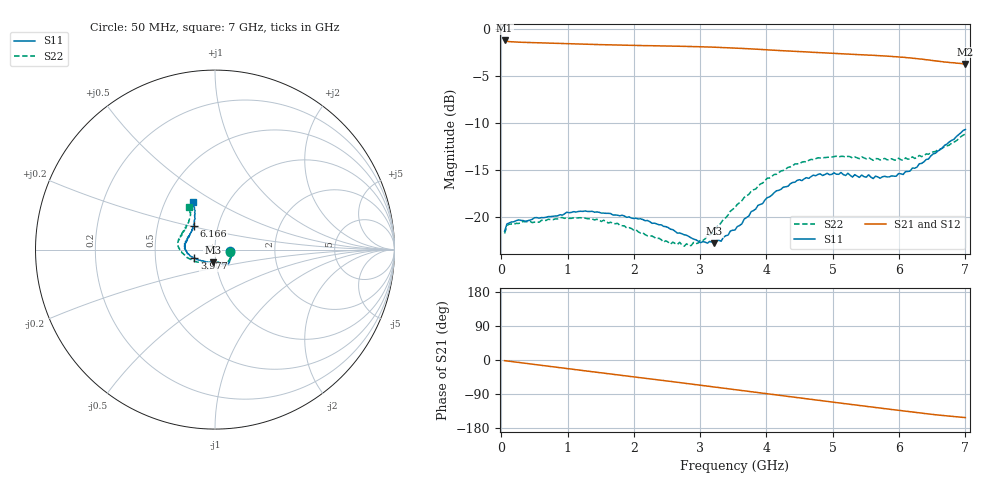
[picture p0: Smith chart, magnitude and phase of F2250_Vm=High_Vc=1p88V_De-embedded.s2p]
! Integrated Device Technology
! Corporate Headquarters
! 6024 Silver Creek Valley Road
! San Jose, CA 95138  USA
! Phone:  1-408-284-8200
! Toll Free:  1-800-223-1366
! Webpage:  http://www.idt.com/
! Timing and RF Division
! 515 Groton Road, Suite 102
! Westford, MA 01886-6024
! Device:  F2250
! Description: Voltage Variable RF Attenuator
! Frequency:  50.0 -  6000.00 MHz
! Package:  3x3 mm Thin QFN Plastic Package: 16 pin
! Ports:  2 RF, 3 DC
!  Pin  1  = GND
!  Pin  2  = NC
!  Pin  3  = RF1  = Port 1
!  Pin  4  = NC
!  Pin  5  = GND
!  Pin  6  = GND
!  Pin  7  = GND
!  Pin  8  = GND
!  Pin  9  = NC
!  Pin 10  = RF2  = Port 2
!  Pin 11  = NC
!  Pin 12  = GND
!  Pin 13  = GND
!  Pin 14  = VCNTRL
!  Pin 15  = VDD
!  Pin 16  = VMODE
! Vcntrl:  1.880 Volts
! Vmode:  +3.300 Volts
! Vdd:  +3.30  Volts
! Current:  1.323 mA
! Data:  The device was measured on a the F2250 evaluation board which has
!  individual transmission lines to the RF pins.  Data was collected
!  using a calibrated network analyzer.  The evaluation board was
!  de-embedded using a TRL calibration technique.
!  The reference plane is the edge of the package pin.
! Misc:  SN 10
!  Action Tracker AT0258
! Date Measured:  2014-11-26
! Date:  2015-10-15  MJV
! Note:
!  Integrated Device Technology supplies this data as a sample of measured
!  data at the package pin for this product.  Your particular data for this
!  product may vary.
!  Data was taken at 25 degrees C.
!  Integrated Device Technology reserves the right to change this data at anytime.
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# GHz S dB R 50
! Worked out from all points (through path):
!   201 points, 50 MHz to 7 GHz, reference 50 ohm
!   highest |S21| = -1.21 dB at 50 MHz (marker M1); lowest = -3.7 dB at 7 GHz (marker M2)
!   group delay of S21, straight-line fit = 61.1 ps
!   lowest |S11| = -22.7 dB at 3.212 GHz (marker M3), VSWR 1.16, Z = 48.2 - j6.95 ohm
!   |S11| at or under -10 dB: start of sweep to end of sweep
!   |S22| runs from -23.1 to -11.1 dB; largest |S21 - S12| = 0.0019
!   S11 on the Smith chart (normalised r, x): 50 MHz: 1.18, -0.02; 3.977 GHz: 0.79, -0.08; 6.166 GHz: 0.76, +0.21; 7 GHz: 0.68, +0.40
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0.05  -21.46 -6.6  -1.21 -1.8  -1.21 -1.8  -21.72 -7.7
0.08475  -20.71 -6.3  -1.30 -2.5  -1.30 -2.5  -20.88 -7.1
0.1195  -20.59 -7.0  -1.33 -3.3  -1.33 -3.3  -20.72 -7.0
0.71025  -19.92 -30.2  -1.48 -16.4  -1.49 -16.5  -20.20 -33.8
1.2315  -19.37 -45.7  -1.60 -27.9  -1.60 -27.9  -20.08 -53.8
1.75275  -19.77 -52.6  -1.70 -39.1  -1.69 -39.1  -20.63 -63.4
2.37825  -20.79 -54.9  -1.78 -52.6  -1.78 -52.7  -22.22 -71.4
2.552  -21.26 -58.6  -1.80 -56.5  -1.80 -56.5  -22.85 -77.9
2.86475  -22.19 -70.2  -1.85 -63.5  -1.85 -63.5  -22.99 -95.2
3.07325  -22.62 -85.9  -1.89 -68.2  -1.89 -68.2  -22.30 -111.4
3.21225  -22.75 -100.3  -1.92 -71.3  -1.92 -71.4  -21.26 -122.6
3.525  -21.34 -129.3  -2.02 -78.4  -2.02 -78.5  -18.95 -141.5
3.97675  -18.15 -157.6  -2.19 -88.6  -2.19 -88.6  -16.10 -162.5
4.4285  -16.27 -172.3  -2.37 -98.6  -2.37 -98.6  -14.33 -177.0
4.7065  -15.52 179.7  -2.47 -104.7  -2.47 -104.7  -13.88 176.6
5.054  -15.42 171.2  -2.60 -112.4  -2.59 -112.4  -13.51 169.0
5.5405  -15.48 155.3  -2.77 -123.1  -2.76 -123.2  -13.65 157.5
5.61  -15.88 154.2  -2.79 -124.5  -2.78 -124.6  -13.94 156.6
5.85325  -15.70 144.2  -2.89 -129.8  -2.89 -129.9  -13.90 149.5
6.166  -15.08 132.1  -3.06 -136.7  -3.07 -136.8  -13.80 140.9
6.54825  -13.19 121.4  -3.37 -144.6  -3.37 -144.7  -13.01 128.6
7  -10.67 115.3  -3.69 -152.0  -3.70 -152.1  -11.15 122.0
